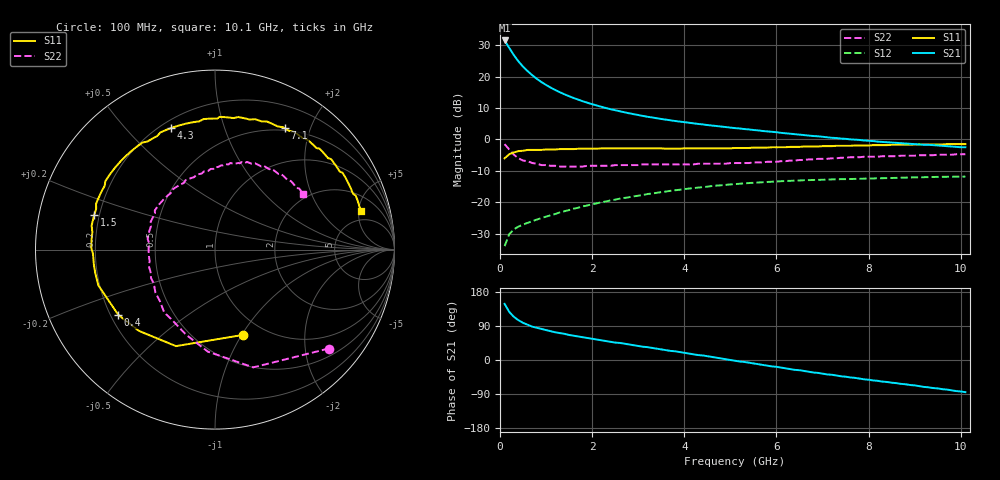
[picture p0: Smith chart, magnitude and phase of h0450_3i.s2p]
!HBFP-0450
!S and NOISE PARAMETERS at Vce=3V  Ic=70mA.  LAST UPDATED  09-04-98
# GHZ S MA R  50
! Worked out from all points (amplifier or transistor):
!   101 points, 100 MHz to 10.1 GHz, reference 50 ohm
!   highest |S21| = 31.5 dB at 100 MHz (marker M1)
!   |S21| within 3 dB of that: start of sweep to 227.8 MHz
!   unconditionally stable (mu >= 1): 2.266 GHz to end of sweep
!   at 1.7 GHz: K = 0.94, MSG = 17.2 dB, |S12| = -21.7 dB
!   at 5.1 GHz: K = 1.08, MAG = 7.2 dB, |S12| = -14.2 dB
!   at 10.1 GHz: K = 1.06, MAG = 3.1 dB, |S12| = -11.8 dB
!   lowest NFmin = 1.98 dB at 1.8 GHz
!   S11 on the Smith chart (normalised r, x): 100 MHz: 0.80, -1.01; 400 MHz: 0.23, -0.29; 1.5 GHz: 0.18, +0.14; 4.3 GHz: 0.24, +0.67; 7.1 GHz: 0.47, +1.63; 10.1 GHz: 3.55, +5.25
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0.1  0.5 -72.0  37.47 148.0  0.02 63.0  0.84 -41.0
0.2  0.58 -112.0  28.55 127.0  0.031 50.0  0.69 -72.0
0.3  0.62 -133.0  21.91 114.0  0.037 44.0  0.57 -94.0
0.4  0.65 -146.0  17.42 105.0  0.041 41.0  0.5 -109.0
0.5  0.66 -156.0  14.33 98.0  0.044 40.0  0.46 -121.0
0.6  0.68 -163.0  12.18 93.0  0.047 39.0  0.45 -129.0
0.7  0.68 -169.0  10.49 88.0  0.05 39.0  0.42 -137.0
0.8  0.68 -173.0  9.18 85.0  0.053 40.0  0.41 -144.0
0.9  0.68 -178.0  8.16 82.0  0.056 40.0  0.39 -151.0
1.1  0.69 175.0  6.66 76.0  0.062 41.0  0.38 -161.0
1.3  0.7 169.0  5.62 71.0  0.069 41.0  0.37 -170.0
1.5  0.7 164.0  4.86 66.0  0.075 41.0  0.37 -177.0
1.8  0.71 157.0  4.03 60.0  0.086 40.0  0.37 174.0
2.1  0.71 150.0  3.46 54.0  0.096 38.0  0.38 167.0
2.5  0.72 142.0  2.91 46.0  0.11 35.0  0.39 158.0
3.5  0.72 124.0  2.11 28.0  0.145 25.0  0.4 140.0
4.3  0.72 110.0  1.76 13.0  0.171 15.0  0.41 126.0
5.1  0.73 95.0  1.51 -2.0  0.194 3.0  0.42 111.0
6.8  0.77 64.0  1.13 -33.0  0.226 -22.0  0.48 81.0
7.1  0.78 60.0  1.08 -38.0  0.229 -26.0  0.49 77.0
8.5  0.82 38.0  0.89 -60.0  0.243 -45.0  0.54 57.0
10.1  0.84 15.0  0.75 -85.0  0.256 -68.0  0.58 32.0
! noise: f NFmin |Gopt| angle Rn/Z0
1.8  1.98  0.65  -149  0.12
2  2.04  0.64  -147  0.14
2.5  2.18  0.65  -137  0.22
3.5  2.48  0.66  -120  0.45
4  2.62  0.69  -110  0.64
5  2.91  0.71  -91  1.11
5.5  3.06  0.74  -82  1.51
7  3.5  0.78  -56  2.91
8  3.79  0.81  -40  4.17
10  4.38  0.82  -12  6.43
